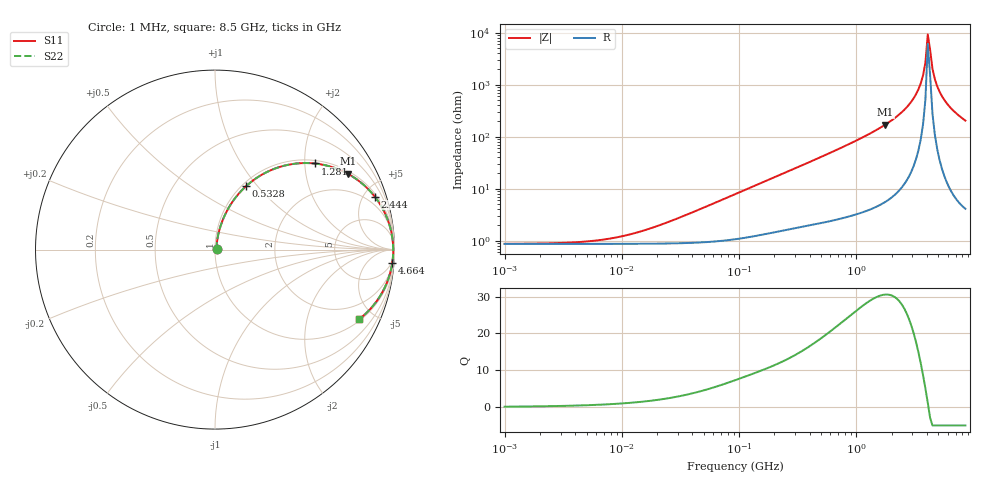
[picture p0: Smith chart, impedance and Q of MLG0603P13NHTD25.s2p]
! S-Parameter Data Generated by TDK Corporation
! Copyright(C) 2025 TDK Corporation.
! All Rights Reserved.
! TDK P/N: MLG0603P13NHTD25 (SMD / SMT Inductor (Coil))
! Property: L=13nH at 500MHz
! Size(LxWxT): 0.6x0.3x0.3mm
! Model Type: s2p (Touchstone File Format Version 1.0)
! Frequency: DC=Yes Start=1MHz Stop=8500MHz 198points Log-sweep
! Model Generated on Feb. 6, 2025
! Terms and conditions regarding TDK Simulation Models:
! 1)This simulation model is being provided solely for informational
!  purposes. Please refer to the specifications of the products in
!  terms of detailed characteristics of such products.
! 2)In no event shall TDK Corporation of any of its subsidiaries be
!  liable for any loss or damage arising, directly or indirectly,
!  from any information contained in this simulation model, including,
!  but not limited to loss or damages arising from any inaccuracies,
!  omissions or errors in connection with such information.
! 3)Any and all copyrights on this simulation model are owned by
!  TDK Corporation.  Duplication or redistribution of this simulation
!  model without prior written permission from TDK Corporation
!  is prohibited.
! 4)This simulation model is subject to any modification or change
!  without any prior notice.
! 5)Neither TDK Corporation nor any of its subsidiaries shall make any
!  warranty, express or implied, including but not limited to the
!  correctness, implied warranties of merchantability and fitness for
!  a particular purpose with respect to this simulation models.
! 6)The use of this simulation model shall be deemed to have consented
!  to the terms and conditions hereof.
! Port Assignments:
!  1 ---@@@--- 2
! Applicable Conditions:
!  Temperature = 25 degC
!  DC Bias Current = 0 A
!  Small Signal Operation
# Hz S MA R 50
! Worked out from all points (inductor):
!   197 points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, 1 MHz to 8.5 GHz, reference 50 ohm
!   read as one part in series: L = 13.5 nH near 31.89 MHz
!   highest Q = 30.5 at 1.769 GHz (marker M1), where L = 15.4 nH
!   self-resonance near 4.061 GHz
!   S11 on the Smith chart (normalised r, x): 1 MHz: 1.02, +0.00; 532.8 MHz: 1.05, +0.87; 1.281 GHz: 1.08, +2.25; 2.444 GHz: 1.21, +5.94; 4.664 GHz: 3, -26; 8.5 GHz: 1.08, -4.07
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1000000  0.008666 5.5  0.9914 -0.0  0.9914 -0.0  0.008666 5.5
4587603  0.009461 24.0  0.9914 -0.2  0.9914 -0.2  0.009461 24.0
1.005548e7  0.01212 44.0  0.9913 -0.5  0.9913 -0.5  0.01212 44.0
2.10461e7  0.0198 62.8  0.9911 -1.0  0.9911 -1.0  0.0198 62.8
9.219544e7  0.07738 77.8  0.9865 -4.4  0.9865 -4.4  0.07738 77.8
4.229561e8  0.3211 67.9  0.9284 -18.7  0.9284 -18.7  0.3211 67.9
5.327649e8  0.3923 64.0  0.8998 -23.1  0.8998 -23.1  0.3923 64.0
8.071757e8  0.5461 54.5  0.8151 -33.1  0.8151 -33.1  0.5461 54.5
1.280704e9  0.7345 40.8  0.6535 -47.2  0.6535 -47.2  0.7345 40.8
1.769233e9  0.8517 29.8  0.497 -58.3  0.497 -58.3  0.8517 29.8
1.940355e9  0.8799 26.5  0.4471 -61.6  0.4471 -61.6  0.8799 26.5
2.444114e9  0.9377 18.4  0.3155 -69.6  0.3155 -69.6  0.9377 18.4
3.07866e9  0.9753 10.2  0.1776 -76.9  0.1776 -76.9  0.9753 10.2
3.535948e9  0.9879 5.3  0.0934 -79.9  0.0934 -79.9  0.9879 5.3
3.703002e9  0.9904 3.7  0.06525 -79.7  0.06525 -79.7  0.9904 3.7
3.877948e9  0.9921 2.1  0.03721 -76.6  0.03721 -76.6  0.9921 2.1
4.061159e9  0.9929 0.5  0.01077 -48.6  0.01077 -48.6  0.9929 0.5
4.453958e9  0.9921 -2.8  0.04911 79.3  0.04911 79.3  0.9921 -2.8
4.664383e9  0.9904 -4.4  0.07733 80.7  0.07733 80.7  0.9904 -4.4
5.115526e9  0.9845 -7.7  0.1339 79.5  0.1339 79.5  0.9845 -7.7
5.87536e9  0.9691 -12.6  0.2186 75.6  0.2186 75.6  0.9691 -12.6
8.5e9  0.8906 -25.9  0.4371 62.9  0.4371 62.9  0.8906 -25.9
